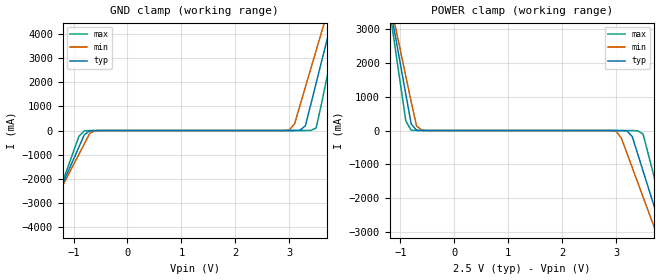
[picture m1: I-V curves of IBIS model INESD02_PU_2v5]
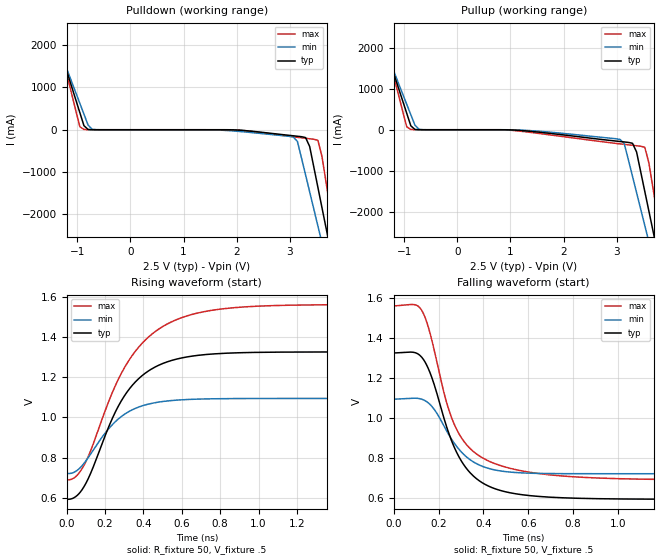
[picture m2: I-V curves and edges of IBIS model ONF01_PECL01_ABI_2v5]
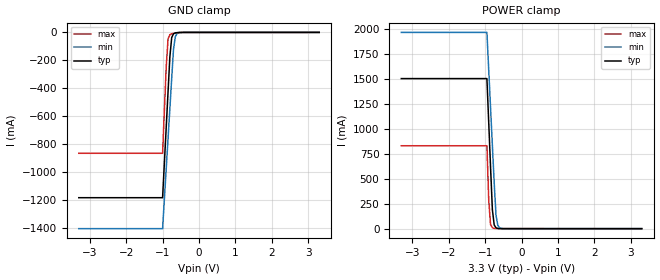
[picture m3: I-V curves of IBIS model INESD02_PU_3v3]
|   This file is an IBIS representation of the   |
|   Integrated Devices Technology, Inc.   |
|   ICS843023I   |
|   FEMTOCLOCKS CRYSTAL-TO-2.5V/3.3V LVPECL CLOCK GENERATOR   |
[IBIS Ver]   4.1
[File name]   843023i.ibs
[File Rev]   1.0
[Date]   30 Dec 2008 | Last modified
|   24 Dec 2008 | Generated
[Source]   Originated at Integrated Devices Technology, Inc.
[Disclaimer]
IDT hereby grants the user of this IBIS model a non-exclusive,
nontransferable license to use this IBIS model under the following terms.
Before using this IBIS model, the user should read this license.
If the user does not accept these terms,  the IBIS model should be
returned to IDT within 30 days.
   The user is granted this license only to use the IBIS model and
is not granted rights to sell, load, rent, lease or license the IBIS
model in whole or in part, or in modified form to anyone other than
user. User may modify the IBIS model to suit its specific
applications but rights to derivative works and such modifications
shall belong to IDT.
   This IBIS model is provided on an "AS IS" basis and IDT makes
absolutely no warranty with respect to the information contained
herein. IDT DISCLAIMS AND CUSTOMER WAIVES ALL WARRANTIES, EXPRESS
OR IMPLIED, INCLUDING WARRANTIES OF MERCHANTABILITY OR FITNESS FOR
A PARTICULAR PURPOSE. The entire risk as to quality and performance
is with the Customer. ACCORDINGLY, IN NO EVENT SHALL THE COMPANY BE
LIABLE FOR ANY DAMAGES, WHETHER IN CONTRACT OR TORT,INCLUDING ANY
LOST PROFITS OR OTHER INCIDENTAL, CONSEQUENTIAL, EXEMPLARY, OR
PUNITIVE DAMAGES ARISING OUT OF THE USE OR APPLICATION OF THE IBIS
model provided in this package. Further, IDT reserves the right to
make changes without notice to any product herein to improve
reliability, function, or design. IDT does not convey any license
under patent rights or any other intellectual property rights,
including those of third parties.
   IDT is not obligated to provide maintenance or support
for the licensed IBIS model.
[Copyright]   Copyright 2004 byIntegrated Devices Technology, Inc.
[Component]   ICS843023I
[Manufacturer] Integrated Devices Technology, Inc.
[Package]
|TSSOP 8 Lead
|   typ   min   max
R_pkg   52.5m   48.8m   56.2m
L_pkg   1.381nH   1.275nH   1.486nH
C_pkg   0.236pF   0.230pF   0.242pF
[Pin]   signal_name   model_name   R_pin   L_pin   C_pin
1   VCC   POWER   56.2m   1.486n   0.242p
2   XTAL_OUT   NC   48.8m   1.275n   0.230p
3   XTAL_IN   NC   48.8m   1.275n   0.230p
4   VEE   GND   56.2m   1.468n   0.242p
5   OE   INESD02_PU   56.2m   1.486n   0.242p
6   VCC   POWER   48.8m   1.275n   0.230p
7   nQ0   ONF01_PECL01_ABI   48.8m   1.275n   0.230p
8   Q   ONF01_PECL01_ABI   56.2m   1.468n   0.242p
[Diff Pin]  inv_pin  vdiff tdelay_typ tdelay_min  tdelay_max
8   7   NA   0  0  0
[Model Selector] INESD02_PU
INESD02_PU_2v5  Buffer selection for 2v5
INESD02_PU_3v3  Buffer selection for 3v3
[Model Selector] ONF01_PECL01_ABI
ONF01_PECL01_ABI_2v5  Buffer selection for 2v5
ONF01_PECL01_ABI_3v3  Buffer selection for 3v3
| Models and submodels in the file (4): INESD02_PU_2v5 (Input), ONF01_PECL01_ABI_2v5 (Output_ECL), INESD02_PU_3v3 (Input), ONF01_PECL01_ABI_3v3 (Output_ECL)
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[Model] INESD02_PU_2v5
Model_type   Input
Polarity   Non-Inverting
Vinl = 1.4V
Vinh = 1.85V
|   typ   min   max
C_comp   2pF   1.5pF   2.5pF
|   typ   min   max
[Voltage range]  2.5V   2.375V   2.625V
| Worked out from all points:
|   GND clamp passes 1 mA (typ) near -0.55 V on its own axis
|   POWER clamp passes 1 mA (typ) near -0.61 V on its own axis
[GND_clamp]
|Voltage   I(typ)   I(min)   I(max)
-2.5V     -8.775A    -7.892A    -10.18A
-1.6V     -4.218A    -4.001A    -4.586A
-900mV    -678.5mA   -979.4mA   -237.6mA
-800mV    -173.9mA   -548.7mA   -10.88mA
-600mV    -1.682mA   -8.796mA   -960.5uA
3V        79.39uA    17.1mA     7.198uA
3.1V      607uA      273.4mA    11.46uA
3.3V      191.5mA    1.785A     278.5uA
3.5V      1.949A     3.298A     103.5mA
3.7V      3.723A     4.812A     2.189A
3.9V      5.498A     6.327A     4.369A
5V        15.27A     14.67A     16.38A
[POWER_clamp]
|Voltage   I(typ)   I(min)   I(max)
-2.5V     15.27A     13.72A     17.74A
-1.2V     3.723A     3.866A     3.551A
-1.1V     2.836A     3.109A     2.461A
-900mV    1.063A     1.596A     283.3mA
-800mV    191.5mA    840mA      6.139mA
-600mV    607uA      8.789mA    64.82uA
3V        -392uA     -16.42mA   -62.09uA
3.4V      -678.5mA   -1.518A    -7.233mA
3.5V      -1.184A    -1.95A     -99.57mA
3.7V      -2.195A    -2.813A    -1.324A
4V        -3.712A    -4.109A    -3.188A
5V        -8.775A    -8.433A    -9.404A
[Model] ONF01_PECL01_ABI_2v5
Model_type  Output_ECL
Polarity   Non-Inverting
Vmeas = .975
Rref = 50
Cref = 0
Vref = .5
|Variable  typ   min   max
C_comp   2p   1.5p   2.5p
[Voltage Range]   2.5   2.375   2.625
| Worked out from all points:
|   rising waveform, R_fixture 50, V_fixture .5: 20-80 % time 228ps typ, 199ps min, 276ps max; typ from 0.592 V to 1.33 V
|   falling waveform, R_fixture 50, V_fixture .5: 20-80 % time 153ps typ, 140ps min, 156ps max; typ from 1.33 V to 0.592 V
| Open source, no load
|  Voltage   I(typ)   I(min)   I(max)
[Pullup]
-2.5V     6.581A     5.758A     7.966A
-1.572V   2.868A     2.671A     3.219A
-1.418V   2.25A      2.158A     2.429A
-953.6mV  402.1mA    621.9mA    72.14mA
-876.3mV  95.6mA     366.6mA    5.897mA
-721.6mV  951.4uA    9.59mA     751.4uA
3.067V    -287.8mA   -237.7mA   -346mA
3.299V    -330.4mA   -1.134A    -380.1mA
3.531V    -1.506A    -2.34A     -427.9mA
3.686V    -2.47A     -3.144A    -1.427A
3.84V     -3.434A    -3.947A    -2.655A
5V        -10.66A    -9.976A    -11.86A
[Pulldown]
-2.5V     6.581A     5.758A     7.966A
-1.495V   2.559A     2.415A     2.824A
-1.418V   2.25A      2.158A     2.429A
-953.6mV  402.1mA    621.9mA    72.14mA
-876.3mV  95.6mA     366.6mA    5.897mA
-721.6mV  951.4uA    9.59mA     751.4uA
3.067V    -142.9mA   -171.4mA   -166.7mA
3.299V    -185mA     -1.067A    -201.5mA
3.531V    -1.361A    -2.272A    -250mA
3.686V    -2.324A    -3.076A    -1.249A
3.84V     -3.288A    -3.879A    -2.478A
5V        -10.51A    -9.904A    -11.69A
[Ramp]
|   typ   min   max
dV/dt_r   0.586/0.368n   0.299/0.313n   0.698/0.446n
dV/dt_f   0.590/0.258n   0.302/0.226n   0.703/0.290n
R_load =   50.0000
[Rising Waveform]
R_fixture = 50
V_fixture = .5   | VCC_typ - 2V
V_fixture_max = 0.625   | VCC_max - 2V
V_fixture_min = 0.375   | VCC_min - 2V
C_fixture = 0.0p
| Time   typ   min   max
0s        592.5mV    720.8mV    689.3mV
46.2ps    605.5mV    731.1mV    704.8mV
92.4ps    659.4mV    774.5mV    766.4mV
241.5ps   1.003V     967.6mV    1.133V
323.4ps   1.138V     1.029V     1.283V
426.3ps   1.231V     1.066V     1.4V
552.3ps   1.285V     1.084V     1.478V
711.9ps   1.312V     1.092V     1.525V
940.8ps   1.323V     1.094V     1.551V
1.999ns   1.326V     1.094V     1.562V
[Falling Waveform]
R_fixture = 50
V_fixture = .5   | VCC_typ - 2V
V_fixture_max = 0.625   | VCC_max - 2V
V_fixture_min = 0.375   | VCC_min - 2V
C_fixture = 0.0p
| Time   typ   min   max
0s        1.326V     1.094V     1.562V
92.4ps    1.328V     1.099V     1.568V
123.9ps   1.306V     1.095V     1.541V
168ps     1.209V     1.061V     1.4V
231ps     973.8mV    945.4mV    1.097V
277.2ps   835.9mV    862.7mV    951mV
348.6ps   716.5mV    784.8mV    838.7mV
447.3ps   647.2mV    740.6mV    773mV
865.2ps   596.5mV    720.8mV    701.4mV
1.999ns   592.4mV    720.7mV    689.3mV
[Model] INESD02_PU_3v3
Model_type   Input
Polarity   Non-Inverting
Vinl = 0.80V
Vinh = 2.0V
|   typ   min   max
C_comp   2pF   1.5pF   2.5pF
|   typ   min   max
[Voltage range]  3.3V   3.15V   3.45V
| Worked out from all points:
|   GND clamp passes 1 mA (typ) near -0.56 V on its own axis
|   POWER clamp passes 1 mA (typ) near -0.61 V on its own axis
[GND_clamp]
|Voltage   I(typ)   I(min)   I(max)
-3.3V     -1.184A    -1.405A    -865.6mA
-1V       -1.184A    -1.405A    -865.6mA
-900mV    -678.5mA   -975.1mA   -244.1mA
-850mV    -426.2mA   -760.2mA   -46.92mA
-800mV    -174mA     -545.4mA   -16.17mA
-750mV    -37.03mA   -330.8mA   -9.981mA
-700mV    -9.767mA   -120.3mA   -7.122mA
-650mV    -3.616mA   -29.78mA   -4.922mA
-600mV    -1.7mA     -7.594mA   -3.115mA
-400mV    -123.9uA   -126uA     -173.9uA
3.3V      1.866nA    3.949uA    0A
[POWER_clamp]
|Voltage   I(typ)   I(min)   I(max)
-3.3V     1.506A     1.97A      832.1mA
-950mV    1.506A     1.97A      832.1mA
-900mV    1.063A     1.592A     287.2mA
-850mV    620.4mA    1.215A     41.77mA
-800mV    191.5mA    837.4mA    8.692mA
-750mV    37.69mA    460.1mA    3.262mA
-700mV    8.032mA    133.8mA    1.662mA
-650mV    2.005mA    32.58mA    840.1uA
-600mV    607uA      8.009mA    378.6uA
-450mV    33.11uA    139.8uA    23.88uA
3.3V      -71.13uA   -77.46uA   -62.11uA
